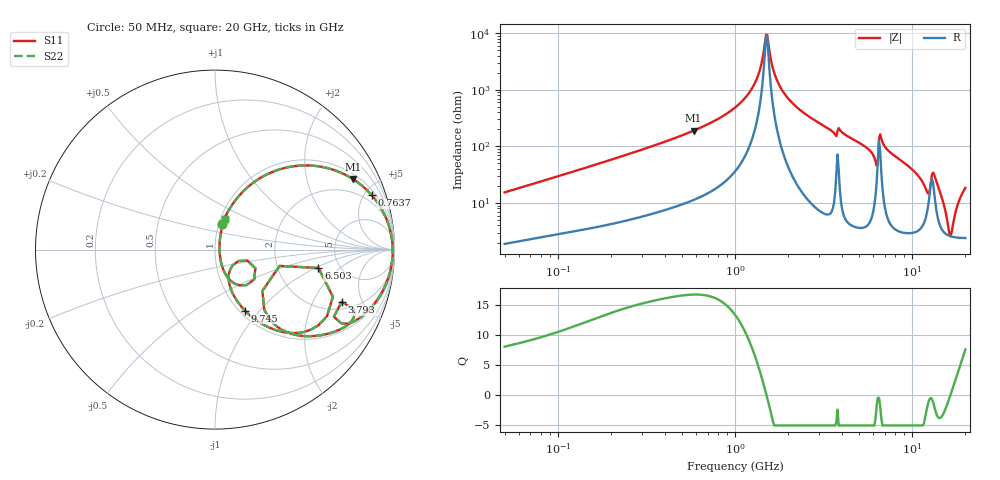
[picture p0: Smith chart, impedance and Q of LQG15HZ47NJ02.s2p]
!Murata Part Number: LQG15HZ47NJ02
!These Parameters are Measured in Series Mode Connection
!  o--[Z]--o
!Port1  Port2
!  o-------o
!Freq. Start=50[MHz] Stop=20[GHz], 401[Steps]
# Hz S RI R 50
!Freq.(Hz) S11(Real) S11(Imag) S21(Real) S21(Imag) S12(Real) S12(Imag) S22(Real) S22(Imag)
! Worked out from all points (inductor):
!   401 points, 50 MHz to 20 GHz, reference 50 ohm
!   read as one part in series: L = 47.8 nH near 51.52 MHz
!   highest Q = 16.7 at 583.2 MHz (marker M1), where L = 51.5 nH
!   self-resonance near 1.498 GHz
!   S11 on the Smith chart (normalised r, x): 50 MHz: 1.04, +0.31; 763.7 MHz: 1.35, +5.61; 3.793 GHz: 2.44, -3.40; 6.503 GHz: 3.46, -1.08; 9.745 GHz: 1.06, -0.84; 20 GHz: 1.05, +0.37
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5e7  0.0401 0.1438  0.9599 -0.1438  0.9599 -0.1438  0.0401 0.1438
1.364002e8  0.1572 0.3245  0.8428 -0.3245  0.8428 -0.3245  0.1572 0.3245
3.721004e8  0.5486 0.4672  0.4514 -0.4672  0.4514 -0.4672  0.5486 0.4672
5.831961e8  0.7682 0.3932  0.2318 -0.3932  0.2318 -0.3932  0.7682 0.3932
7.636728e8  0.873 0.3036  0.127 -0.3036  0.127 -0.3036  0.873 0.3036
1e9  0.9459 0.192  0.0541 -0.192  0.0541 -0.192  0.9459 0.192
1.289994e9  0.9829 0.0749  0.0171 -0.0749  0.0171 -0.0749  0.9829 0.0749
1.498439e9  0.99 0.00306  0.00997 -0.00306  0.00997 -0.00306  0.99 0.00306
1.689197e9  0.9877 -0.0553  0.0123 0.0553  0.0123 0.0553  0.9877 -0.0553
1.848039e9  0.9811 -0.0993  0.0189 0.0993  0.0189 0.0993  0.9811 -0.0993
2.728004e9  0.8981 -0.2877  0.1019 0.2877  0.1019 0.2877  0.8981 -0.2877
3.792786e9  0.7059 -0.2911  0.2941 0.2911  0.2941 0.2911  0.7059 -0.2911
5.598765e9  0.4603 -0.4771  0.5397 0.4771  0.5397 0.4771  0.4603 -0.4771
6.217679e9  0.2745 -0.3353  0.7255 0.3353  0.7255 0.3353  0.2745 -0.3353
6.503449e9  0.5766 -0.1026  0.4234 0.1026  0.4234 0.1026  0.5766 -0.1026
6.701223e9  0.6241 -0.3709  0.3759 0.3709  0.3759 0.3709  0.6241 -0.3709
7.442007e9  0.4001 -0.4627  0.5999 0.4627  0.5999 0.4627  0.4001 -0.4627
9.745021e9  0.1674 -0.3402  0.8326 0.3402  0.8326 0.3402  0.1674 -0.3402
1.220001e10  0.0828 -0.1148  0.9172 0.1148  0.9172 0.1148  0.0828 -0.1148
1.354865e10  0.1349 -0.1991  0.8651 0.1991  0.8651 0.1991  0.1349 -0.1991
1.646126e10  0.0252 0.000816  0.9748 -0.000816  0.9748 -0.000816  0.0252 0.000816
2e10  0.0536 0.169  0.9464 -0.169  0.9464 -0.169  0.0536 0.169
